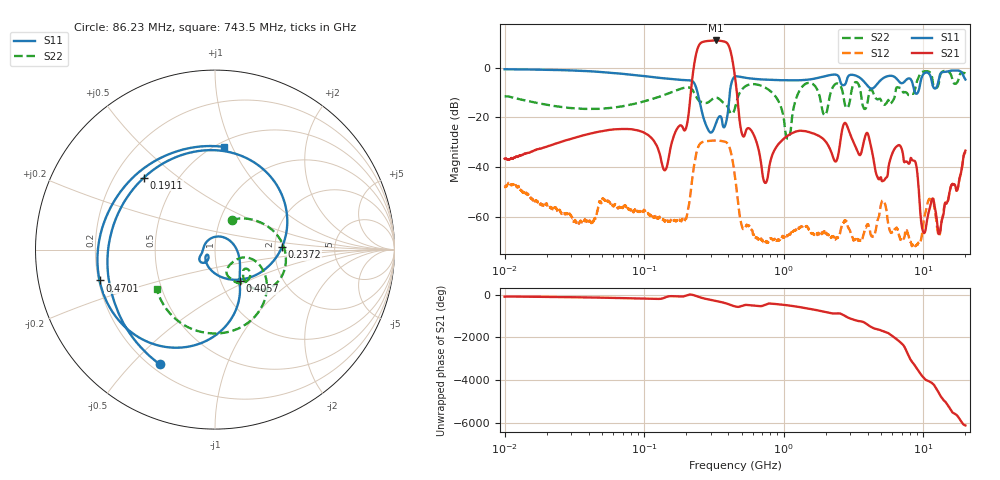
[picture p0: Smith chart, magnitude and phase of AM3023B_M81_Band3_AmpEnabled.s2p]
!Agilent Technologies,E8364B,MY43040894,A.07.50.67
!Agilent E8364B: A.07.50.67
!Date: Tuesday, October 27, 2020 10:43:26
!Correction: S11(Full 2 Port(1,2))
!S21(Full 2 Port(1,2))
!S12(Full 2 Port(1,2))
!S22(Full 2 Port(1,2))
!S2P File: Measurements: S11, S21, S12, S22:Log Frequency Sweep
# Hz S  dB  R 50
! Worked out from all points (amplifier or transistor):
!   3201 points, 10 MHz to 20 GHz, reference 50 ohm
!   highest |S21| = 10.9 dB at 325.3 MHz (marker M1)
!   |S21| within 3 dB of that: 242.1 MHz to 408.9 MHz (166.8 MHz wide, 51.3 % of centre)
!   unconditionally stable (mu >= 1): start of sweep to end of sweep
!   at 35.47 MHz: K = 3626.37, MAG = -21.3 dB, |S12| = -61.9 dB
!   at 447.2 MHz: K = 65.07, MAG = -1.2 dB, |S12| = -43.7 dB
!   at 20 GHz: K = 313.80, MAG = -27.7 dB, |S12| = -33.8 dB
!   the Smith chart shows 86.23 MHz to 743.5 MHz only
!   S11 on the Smith chart (normalised r, x): 86.23 MHz: 0.23, -0.60; 191.1 MHz: 0.32, +0.38; 237.2 MHz: 2.19, +0.08; 405.7 MHz: 1.22, -0.46; 470.1 MHz: 0.20, -0.13; 743.5 MHz: 0.55, +0.93
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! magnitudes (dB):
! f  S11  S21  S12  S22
! 10 MHz  -0.6  -36.6  -47.9  -11.5
! 35.55 MHz  -1.3  -27.4  -61.8  -16.5
! 86.23 MHz  -3.0  -25.0  -57.2  -14.5
! 126.1 MHz  -4.0  -32.8  -60.5  -11.8
! 191.1 MHz  -5.0  -24.7  -61.2  -8.2
! 237.2 MHz  -8.5  6.3  -34.0  -12.0
! 325.3 MHz  -22.6  10.9  -29.2  -12.0
! 405.7 MHz  -13.0  8.5  -31.6  -17.2
! 447.2 MHz  -3.6  -3.8  -43.7  -16.1
! 470.1 MHz  -3.5  -14.7  -53.7  -11.6
! 743.5 MHz  -4.8  -46.3  -69.9  -8.1
! 1.072 GHz  -5.1  -27.3  -67.4  -28.5
! 1.59 GHz  -4.6  -26.3  -66.5  -6.3
! 1.96 GHz  -3.5  -29.2  -66.0  -19.1
! 2.392 GHz  -2.9  -37.3  -68.2  -6.3
! 2.759 GHz  -6.6  -22.2  -61.7  -15.4
! 5.639 GHz  -3.3  -39.6  -63.3  -13.2
! 8.525 GHz  -8.4  -37.4  -71.6  -10.3
! 9.972 GHz  -2.7  -66.0  -63.3  -1.6
! 11.36 GHz  -4.3  -54.3  -53.4  -2.6
! 13.01 GHz  -3.7  -66.6  -67.4  -4.8
! 20 GHz  -4.8  -33.3  -33.8  -2.3
